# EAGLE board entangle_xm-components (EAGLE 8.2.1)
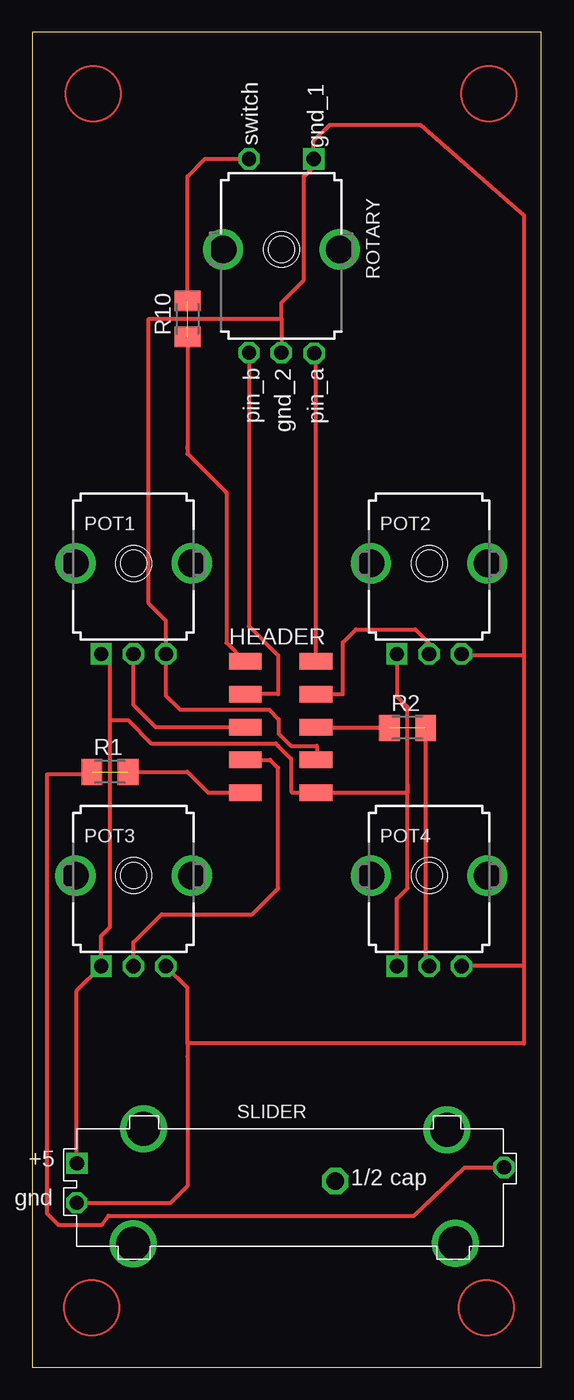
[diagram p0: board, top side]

Size 39.35 x 103.14 mm. Coordinates in mm from the lower left corner, seen from the top.
Outline: 0,0 39.35,0 39.35,103.14 0,103.14 0,0
Copper layers (1*16): Top 0.035mm / dielectric 1.5mm / Bottom 0.035mm
Design rules "default *": minimum track width 6mil, minimum drill 0.35mm, track to track 16mil, track to pad 16mil, pad to pad 16mil, via to via 16mil, smd to smd 16mil, copper to edge 40mil, drill to drill 6mil, minimum pad ring 10mil, minimum via ring 8mil, stop-mask expansion 4mil, vias tented up to drill 0mil, thermal gap 10mil

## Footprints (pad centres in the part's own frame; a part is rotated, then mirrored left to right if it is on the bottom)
2X05SMD = smd 2.54 x 1.27: 1 -2.54,2.54; 2 2.92,2.54; 3 -2.54,0; 4 2.92,0; 5 -2.54,-2.54; 6 2.92,-2.54; 7 -2.54,-5.08; 8 2.92,-5.08; 9 -2.54,-7.62; 10 2.92,-7.62
9MM_SNAP-IN_POT = drill 1.1 square: 1 -2.5,-7 | drill 1.1 octagon: 2 0,-7; 3 2.5,-7 | drill 2.1 pad 2.794: .1 -4.5,0; .2 4.5,0
M1206 = smd 1.6 x 2: 1 -1.4,0; 2 1.4,0
ROTARY_ENCODER = drill 1.1 square: 1 -7,2.5 | drill 1.1 octagon: 2 -7,-2.5; 3 8.019,2.548; 4 7.97,0; 5 7.97,-2.5 | drill 2.1 pad 2.794: .1 0,4.5; .2 0,-4.5
CENTER_DETENT_SLIDER = drill 1.1 square: 1 -17.98,1.896 | drill 1.1 octagon: 2 -17.996,-1.148; 3 15.054,1.584 | drill 1.354 octagon: 4 2.004,0.522 | drill 2.608 pad 3.302: .1 -12.828,4.555; .2 10.641,4.495; .3 -13.628,-4.325; .4 11.281,-4.285

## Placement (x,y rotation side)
HEADER  PINHD-2X5-SMD  [2X05SMD]  19,52 0 top
POT1  [9MM_SNAP-IN_POT]  7.82,62.11 0 top
POT2  [9MM_SNAP-IN_POT]  30.68,62.11 0 top
POT3  [9MM_SNAP-IN_POT]  7.82,37.98 0 top
POT4  [9MM_SNAP-IN_POT]  30.68,37.98 0 top
R1  0  [M1206]  6,46 0 top
R2  0  [M1206]  29,49.4 0 top
R10  0  [M1206]  12,81 90 top
ROTARY  ROTARY_ENCODER  [ROTARY_ENCODER]  19.25,86.37 270 top
SLIDER  CENTER_DETENT_SLIDER  [CENTER_DETENT_SLIDER]  21.42,13.85 0 top

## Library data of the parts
HEADER = fab
POT1-POT4 = MusicThingModular
R1 R2 R10 = rcl
ROTARY SLIDER = mcetilia

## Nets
GND: HEADER.8 POT1.3 POT2.3 POT3.3 POT4.3 ROTARY.1 ROTARY.4 SLIDER.2
PIN_A: HEADER.2 ROTARY.3
PIN_B: HEADER.3 ROTARY.5
POT1: HEADER.5 POT1.2
POT2: HEADER.4 POT2.2
POT3: HEADER.7 POT3.2
POT4: HEADER.6 POT4.2 R2.1 R2.2
SLIDER: HEADER.9 R1.1 R1.2 SLIDER.3
SWITCH: HEADER.1 R10.1 R10.2 ROTARY.2
VCC: HEADER.10 POT1.1 POT2.1 POT3.1 POT4.1 SLIDER.1

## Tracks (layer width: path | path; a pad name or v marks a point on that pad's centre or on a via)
GND
  Top 0.305: 38,55 38,89 30,96 23,96 21.75,94.75 ROTARY.1 21.75,93.25 22,93 21,92 21,84 19.25,82.25 19.25,81 | 38,55 33.29,55 | 38,55 38,31.02 | 19.25,81 ROTARY.4 | SLIDER.2 10.7,12.7 12,14 12,24 12,25 | POT3.3 12,29.3 12,25 | 38,31.02 38,25 12,25 | 10,81 13,81 19.25,81 | 10,81 11,81 | 10,81 9,81 9,59 10.32,57.68 POT1.3 10.32,51.91 11.43,50.8 18.3,50.8 19.05,50.05 19.05,48.96 20,48 22,48 | HEADER.8 22,47 HEADER.8 | 38,31.02 35.56,31.02 33.22,31.02 33.2,31 | 22,48 | 22,48 22,47 HEADER.8
  Top 0.406: POT2.3 33.29,55 | 33.2,31 POT4.3 | 21.96,46.96 HEADER.8
PIN_A
  Top 0.305: HEADER.2 21.92,78.23
  Top 0.406: 21.92,78.23 ROTARY.3
PIN_B
  Top 0.305: HEADER.3 19,52 19,55 16.75,57.25 ROTARY.5
POT1
  Top 0.305: HEADER.5 9.54,49.46 7.8,51.2 7.8,55.09
  Top 0.406: POT1.2 7.8,55.09
POT2
  Top 0.305: HEADER.4 24,52 24,56 25,57 29.6,57 30.7,55.9 30.7,55.13 POT2.2
  Top 0.406: POT2.2 30.7,55.13
POT3
  Top 0.305: HEADER.7 18.38,46.92 19,46.3 19,37 17,35 10,35 7.82,32.82 POT3.2 7.8,31
  Top 0.406: 7.8,31 POT3.2
POT4  (1 unrouted)
  Top 0.305: R2.2 30.4,31.26 | R2.1 21.98,49.4
  Top 0.406: 30.4,31.26 POT4.2 | 21.98,49.4 HEADER.6
SLIDER  (1 unrouted)
  Top 0.305: R1.2 12,46 13.6,44.4 16.44,44.4 HEADER.9 | SLIDER.3 33.43,15.43 29.5,11.7 5.9,11.7 5.4,11 2,11 1.17,11.83 1.17,45.83 4.43,45.83 R1.1
SWITCH  (1 unrouted)
  Top 0.305: R10.1 12,71.12 | 12,71.12 12,71 | 12,71.12 12,70.58 15.01,67.56 15.01,55.99 HEADER.1 | R10.2 12,92 13.37,93.37 ROTARY.2
VCC
  Top 0.305: 6,50 6,49 6,46 6,34 5.5,33.5 5.32,33.32 POT3.1 3.44,29.1 SLIDER.1 | 6,50 6,54.43 POT1.1 | POT2.1 28.18,51.82 29,51 29,45 | 29,45 29,44.4 21.94,44.4 | 21.94,44.4 HEADER.10 | POT4.1 28.18,36.18 29,37 29,45 | 21.94,44.4 20.1,44.4 20,44.5 20,47 19,48 | 6,50 7.4,50 9.2,48.2 18.8,48.2 19,48 | 19,48 19.24,47.76
  Top 0.406: POT1.1
(copper drawn outside any net)
  shapes: Top circle x4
